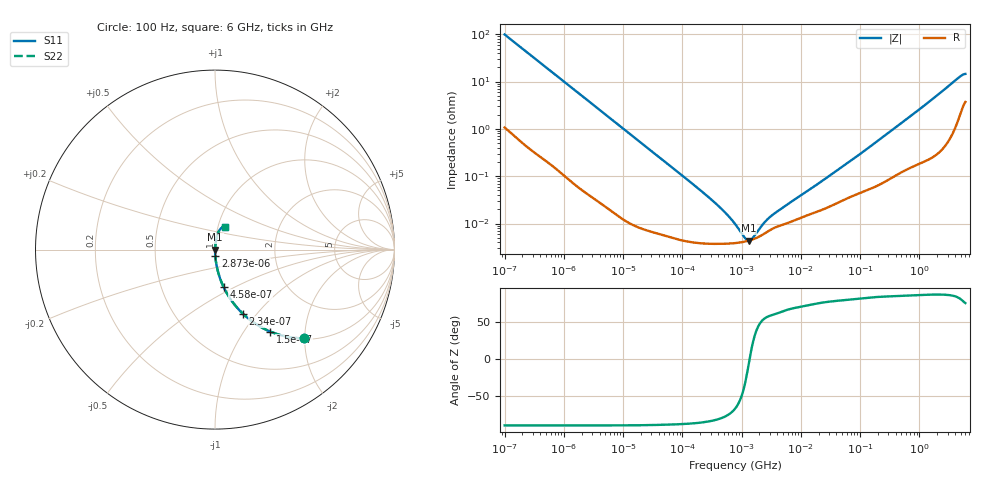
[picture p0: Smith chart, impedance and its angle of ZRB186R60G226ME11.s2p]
!Murata Part Number: ZRB186R60G226ME11
!These Parameters are Measured in Series Mode Connection
!Data Generated on Jun 10, 2025
!  o--ll--o
!Port1  Port2
!  o------o
!Operation Temp=25[degC], DC Bias Voltage=0[V]
!Freq. Start=100[Hz] Stop=6[GHz] 401[Steps]
# Hz S RI R 50
!Freq.(Hz) S11(Real) S11(Imag) S21(Real) S21(Imag) S12(Real) S12(Imag) S22(Real) S22(Imag)
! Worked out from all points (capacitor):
!   401 points, 100 Hz to 6 GHz, reference 50 ohm
!   read as one part in series: C = 16 uF near 109 Hz
!   lowest |Z| = 4.37 mohm at 1.326 MHz (marker M1)
!   series resonance near 1.368 MHz, so ESL is about 840 pH
!   S11 on the Smith chart (normalised r, x): 100 Hz: 1.02, -1.98; 150 Hz: 1.01, -1.33; 234 Hz: 1.01, -0.85; 458 Hz: 1.00, -0.44; 2.873 kHz: 1.00, -0.07; 6 GHz: 1.07, +0.28
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100  0.4952 -0.4946  0.5048 0.4946  0.5048 0.4946  0.4952 -0.4946
150  0.3078 -0.4564  0.6922 0.4564  0.6922 0.4564  0.3078 -0.4564
234  0.1558 -0.3577  0.8442 0.3577  0.8442 0.3577  0.1558 -0.3577
320  0.0908 -0.2824  0.9092 0.2824  0.9092 0.2824  0.0908 -0.2824
458  0.0474 -0.2074  0.9526 0.2074  0.9526 0.2074  0.0474 -0.2074
897  0.0135 -0.1104  0.9865 0.1104  0.9865 0.1104  0.0135 -0.1104
2008  0.00303 -0.0501  0.997 0.0501  0.997 0.0501  0.00303 -0.0501
2873  0.00161 -0.0351  0.9984 0.0351  0.9984 0.0351  0.00161 -0.0351
40335  6.65e-05 -0.00254  0.9999 0.00254  0.9999 0.00254  6.65e-05 -0.00254
289253  3.74e-05 -0.000342  1 0.000342  1 0.000342  3.74e-05 -0.000342
452617  3.72e-05 -0.000204  1 0.000204  1 0.000204  3.72e-05 -0.000204
774597  3.85e-05 -9.05e-05  1 9.05e-05  1 9.05e-05  3.85e-05 -9.05e-05
1325623  4.34e-05 -4.7e-06  1 4.7e-06  1 4.7e-06  4.34e-05 -4.7e-06
2169299  5.62e-05 6.85e-05  0.9999 -6.85e-05  0.9999 -6.85e-05  5.62e-05 6.85e-05
2372521  6.01e-05 8.19e-05  0.9999 -8.19e-05  0.9999 -8.19e-05  6.01e-05 8.19e-05
3712478  8.28e-05 0.000146  0.9999 -0.000146  0.9999 -0.000146  8.28e-05 0.000146
1.555665e7  0.000163 0.000545  0.9998 -0.000545  0.9998 -0.000545  0.000163 0.000545
8.527865e7  0.000414 0.00252  0.9996 -0.00252  0.9996 -0.00252  0.000414 0.00252
3.124326e8  0.000934 0.00852  0.9991 -0.00852  0.9991 -0.00852  0.000934 0.00852
1.565993e9  0.00396 0.0397  0.996 -0.0397  0.996 -0.0397  0.00396 0.0397
4.586474e9  0.0291 0.1143  0.9709 -0.1143  0.9709 -0.1143  0.0291 0.1143
6e9  0.0532 0.1283  0.9468 -0.1283  0.9468 -0.1283  0.0532 0.1283
